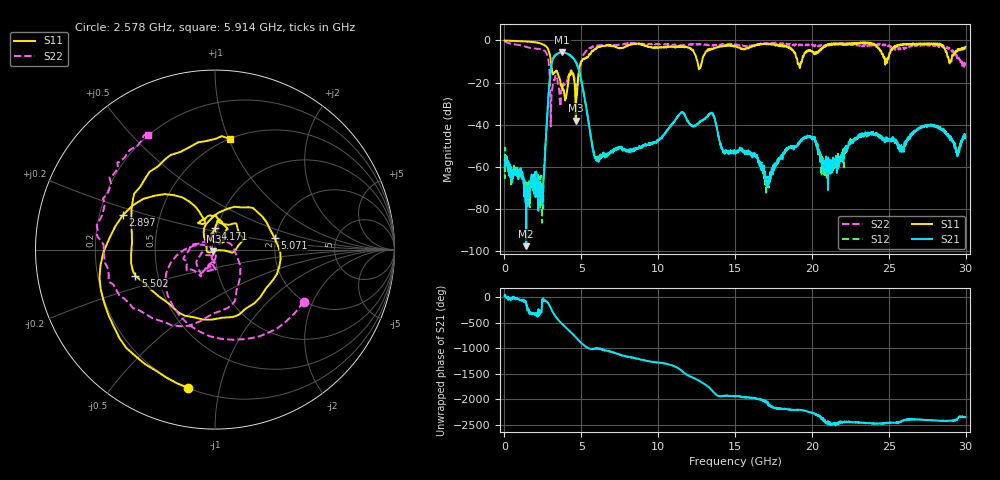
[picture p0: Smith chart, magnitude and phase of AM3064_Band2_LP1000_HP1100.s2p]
# Hz S DB R 50.0
!freq dBS11 angS11 dBS21 angS21 dBS12 angS12 dBS22 angS22
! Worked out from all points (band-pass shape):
!   1600 points, 10 MHz to 29.98 GHz, reference 50 ohm
!   highest |S21| = -5.65 dB at 3.759 GHz (marker M1); lowest = -97.6 dB at 1.416 GHz (marker M2)
!   |S21| within 3 dB of the highest: 3.161 GHz to 4.506 GHz (1.346 GHz wide, 35.1 % of centre)
!   lowest |S11| = -38.0 dB at 4.64 GHz (marker M3), VSWR 1.03, Z = 49.2 - j0.916 ohm
!   |S11| at or under -10 dB: 3.021 GHz to 4.998 GHz (1.977 GHz wide, 49.3 % of centre); 12.56 GHz to 12.85 GHz (288.6 MHz wide, 2.27 % of centre); 19.06 GHz to 19.34 GHz (285.3 MHz wide, 1.49 % of centre)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
!   |S22| runs from -40.8 to -0.2 dB; largest |S21 - S12| = 0.018
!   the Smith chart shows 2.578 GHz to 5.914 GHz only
!   S11 on the Smith chart (normalised r, x): 2.578 GHz: 0.20, -0.81; 2.897 GHz: 0.30, +0.17; 4.171 GHz: 0.97, +0.23; 5.071 GHz: 1.96, +0.29; 5.502 GHz: 0.37, -0.14; 5.914 GHz: 0.50, +1.01
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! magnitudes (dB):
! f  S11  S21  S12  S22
! 10 MHz  0.0  -56.7  -58.8  -0.2
! 1.416 GHz  -0.5  -97.6  -69.2  -3.0
! 2.372 GHz  -1.4  -70.8  -73.0  -4.2
! 2.578 GHz  -2.1  -63.3  -61.7  -4.8
! 2.897 GHz  -5.2  -22.8  -22.7  -11.6
! 3.159 GHz  -16.1  -8.7  -8.7  -20.7
! 3.759 GHz  -22.0  -5.7  -5.8  -22.8
! 4.171 GHz  -18.6  -6.7  -6.5  -15.9
! 4.64 GHz  -38.0  -10.2  -10.3  -21.7
! 5.015 GHz  -9.9  -19.6  -19.6  -9.6
! 5.071 GHz  -9.4  -21.8  -21.8  -8.4
! 5.502 GHz  -6.6  -40.2  -40.2  -4.1
! 5.914 GHz  -4.1  -56.1  -55.3  -2.6
! 10 GHz  -3.4  -47.4  -47.6  -1.8
! 13.43 GHz  -4.2  -34.3  -34.1  -2.4
! 14.18 GHz  -2.6  -51.5  -51.5  -1.9
! 15 GHz  -2.6  -53.4  -52.6  -1.8
! 17.1 GHz  -1.7  -67.8  -64.6  -1.4
! 19.99 GHz  -4.9  -46.0  -46.1  -2.0
! 20.95 GHz  -2.6  -60.2  -62.7  -2.1
! 25 GHz  -8.0  -47.3  -46.8  -2.3
! 29.98 GHz  -3.0  -45.6  -45.8  -10.5
